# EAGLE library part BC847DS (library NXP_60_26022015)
NPN/NPN general-purpose transistor pair in a small SOT457 (SC-74) Surface-Mounted Device (SMD) plastic package. AAL Eindhoven MK
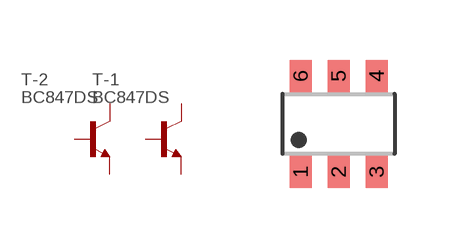
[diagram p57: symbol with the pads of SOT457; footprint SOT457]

Designator prefix T; gates -1=NPN -2=NPN

## BC847DS  [SOT457]
1  -1:E  pas
2  -1:B  pas
3  -2:C  pas
4  -2:E  pas
5  -2:B  pas
6  -1:C  pas

## Footprint SOT457 (pad centres in mm)
SOT457 TSOP6: Plastic surface-mounted package; 6 lead JEIDA: SC73 A.K.A. SOT23-6
smd 0.55 x 0.8: 1 -0.95,-1.2; 2 0,-1.2; 3 0.95,-1.2; 4 0.95,1.2; 5 0,1.2; 6 -0.95,1.2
